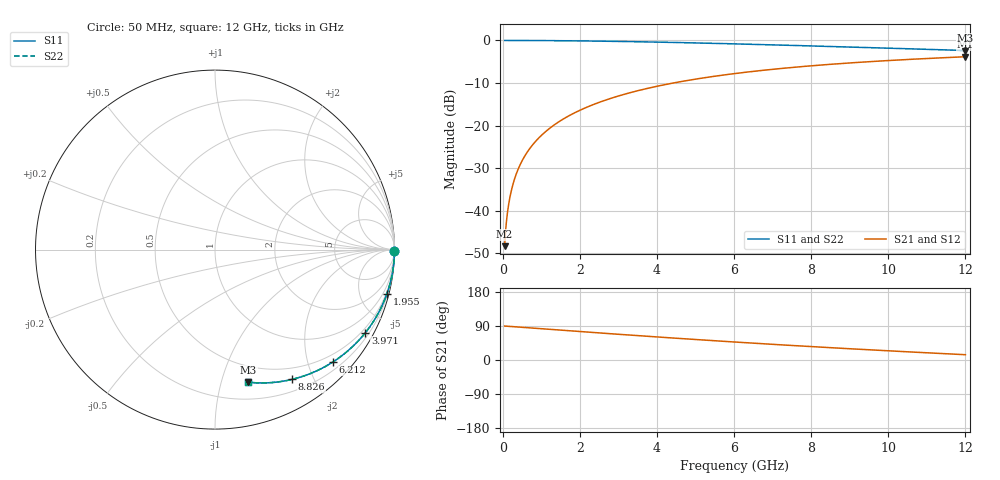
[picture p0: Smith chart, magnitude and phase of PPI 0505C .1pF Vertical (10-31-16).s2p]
# GHz S MA R 50
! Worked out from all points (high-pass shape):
!   1601 points, 50 MHz to 12 GHz, reference 50 ohm
!   highest |S21| = -3.83 dB at 12 GHz (marker M1); lowest = -48.3 dB at 50 MHz (marker M2)
!   |S21| within 3 dB of the highest: 6.947 GHz to end of sweep
!   lowest |S11| = -2.4 dB at 12 GHz (marker M3), VSWR 7.40, Z = 17.4 - j61.2 ohm
!   |S11| at or under -10 dB: nowhere
!   |S22| runs from -2.4 to 0.0 dB; largest |S21 - S12| = 0
!   S11 on the Smith chart (normalised r, x): 50 MHz: open; 1.955 GHz: 0.35, -7.83; 3.971 GHz: 0.35, -3.85; 6.212 GHz: 0.35, -2.45; 8.826 GHz: 0.35, -1.71; 12 GHz: 0.35, -1.22
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0.05  1 -0.4  0.00384 89.6  0.00384 89.6  1 -0.4
0.079875  1 -0.6  0.006134 89.4  0.006134 89.4  1 -0.6
0.1246875  0.9999 -0.9  0.009575 89.1  0.009575 89.1  0.9999 -0.9
0.1545625  0.9999 -1.2  0.01187 88.8  0.01187 88.8  0.9999 -1.2
0.2367188  0.9998 -1.8  0.01817 88.2  0.01817 88.2  0.9998 -1.8
0.2964688  0.9997 -2.2  0.02276 87.8  0.02276 87.8  0.9997 -2.2
0.3711563  0.9996 -2.8  0.02849 87.2  0.02849 87.2  0.9996 -2.8
0.557875  0.999 -4.2  0.04279 85.8  0.04279 85.8  0.999 -4.2
0.8043438  0.998 -6.0  0.06161 84.0  0.06161 84.0  0.998 -6.0
1.118031  0.9963 -8.3  0.08544 81.6  0.08544 81.6  0.9963 -8.3
1.498938  0.9933 -11.2  0.1141 78.8  0.1141 78.8  0.9933 -11.2
1.954531  0.9888 -14.5  0.1479 75.5  0.1479 75.5  0.9888 -14.5
2.044156  0.9878 -15.2  0.1545 74.8  0.1545 74.8  0.9878 -15.2
2.903062  0.9761 -21.4  0.2159 68.6  0.2159 68.6  0.9761 -21.4
3.971094  0.9572 -28.9  0.2878 61.0  0.2878 61.0  0.9572 -28.9
4.038312  0.9559 -29.4  0.2921 60.6  0.2921 60.6  0.9559 -29.4
6.025  0.9116 -42.5  0.4089 47.4  0.4089 47.4  0.9116 -42.5
6.211719  0.9071 -43.7  0.4187 46.2  0.4187 46.2  0.9071 -43.7
8.019156  0.8619 -54.6  0.5045 35.3  0.5045 35.3  0.8619 -54.6
8.825781  0.8413 -59.2  0.5376 30.7  0.5376 30.7  0.8413 -59.2
10.01331  0.8113 -65.7  0.5814 24.2  0.5814 24.2  0.8113 -65.7
12  0.762 -75.8  0.6437 13.9  0.6437 13.9  0.762 -75.8
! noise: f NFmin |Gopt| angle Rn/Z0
0.05  0.007396  0.9962  0.3735  0.4435
1.372  0.008794  0.9017  9.219  0.01946
2.701  0.01057  0.8242  16.14  0.01238
4.031  0.01242  0.7644  21.73  0.01033
5.36  0.01429  0.7188  26.52  0.009544
6.682  0.01617  0.6842  30.76  0.009256
8.012  0.01809  0.6575  34.68  0.009224
9.341  0.02005  0.6373  38.34  0.009352
10.67  0.02207  0.6221  41.8  0.009596
12  0.02417  0.6111  45.07  0.009936
